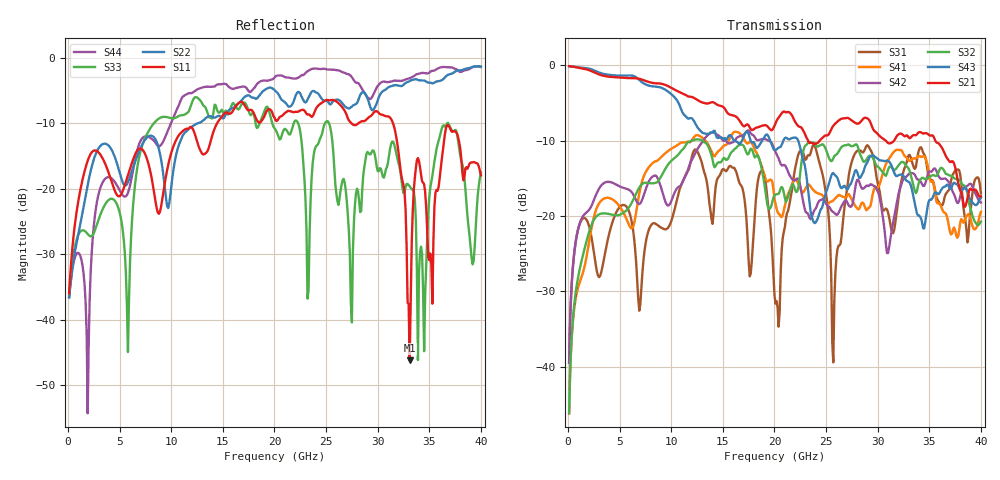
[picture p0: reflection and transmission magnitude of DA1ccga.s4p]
! ADC12DJ3200QML-SP
! 196-pin NWE package
! CCGA Ceramic Package with columns (ceramic column grid array)
! Texas Instruments 4/21/2021
! Single-ended  S-parameters
! PORT#  PORT_NAME  NET_NAME
! PORT1:  DAxN.DIEBUMP DAxN
! PORT2:  DAxN.BGA  DAxN
! PORT3:  DAxP.DIEBUMP DAxP
! PORT4:  DAxP.BGA  DAxP
! Touchstone Ver. 1.0
! Number of ports is 4
# Hz	S	MA	R	50.000000
! SCATTERING PARAMETERS  :
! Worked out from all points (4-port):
!   400 points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, 100 MHz to 40 GHz, reference 50 ohm
!   strongest paths, dB at 100 MHz, 10.1 GHz, 20.1 GHz, 30.1 GHz, 40 GHz:
!     S21: -0.1, -3.1, -7.7, -9.3, -17.4
!     S43: -0.1, -4.0, -11.2, -12.5, -17.5
!     S32: -46.2, -12.5, -17.1, -13.5, -20.8
!     S42: -39.5, -17.7, -11.5, -17.1, -18.2
!     S41: -46.2, -11.0, -18.4, -16.1, -19.4
!     S31: -39.5, -20.2, -31.6, -16.2, -17.0
!   lowest |S11| = -46.2 dB at 33.1 GHz (marker M1), VSWR 1.01, Z = 49.9 + j0.478 ohm
!   |S11| at or under -10 dB: start of sweep to 14.44 GHz; 27.45 GHz to 28.13 GHz (677.8 MHz wide, 2.44 % of centre); 31.48 GHz to end of sweep
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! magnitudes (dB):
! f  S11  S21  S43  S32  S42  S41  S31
! 100 MHz  -36.0  -0.1  -0.1  -46.2  -39.5  -46.2  -39.5
! 23.8 GHz  -8.6  -10.4  -20.8  -10.3  -19.4  -16.6  -10.6
! 25.7 GHz  -6.5  -8.0  -14.3  -12.3  -19.5  -17.9  -39.4
! 31.6 GHz  -10.6  -10.0  -14.2  -13.9  -20.1  -11.4  -21.8
! 33.1 GHz  -46.2  -9.7  -15.6  -14.0  -14.4  -12.7  -11.9
! 33.8 GHz  -15.6  -9.2  -19.6  -16.7  -15.1  -12.2  -12.6
! 40 GHz  -17.9  -17.4  -17.5  -20.8  -18.2  -19.4  -17.0
